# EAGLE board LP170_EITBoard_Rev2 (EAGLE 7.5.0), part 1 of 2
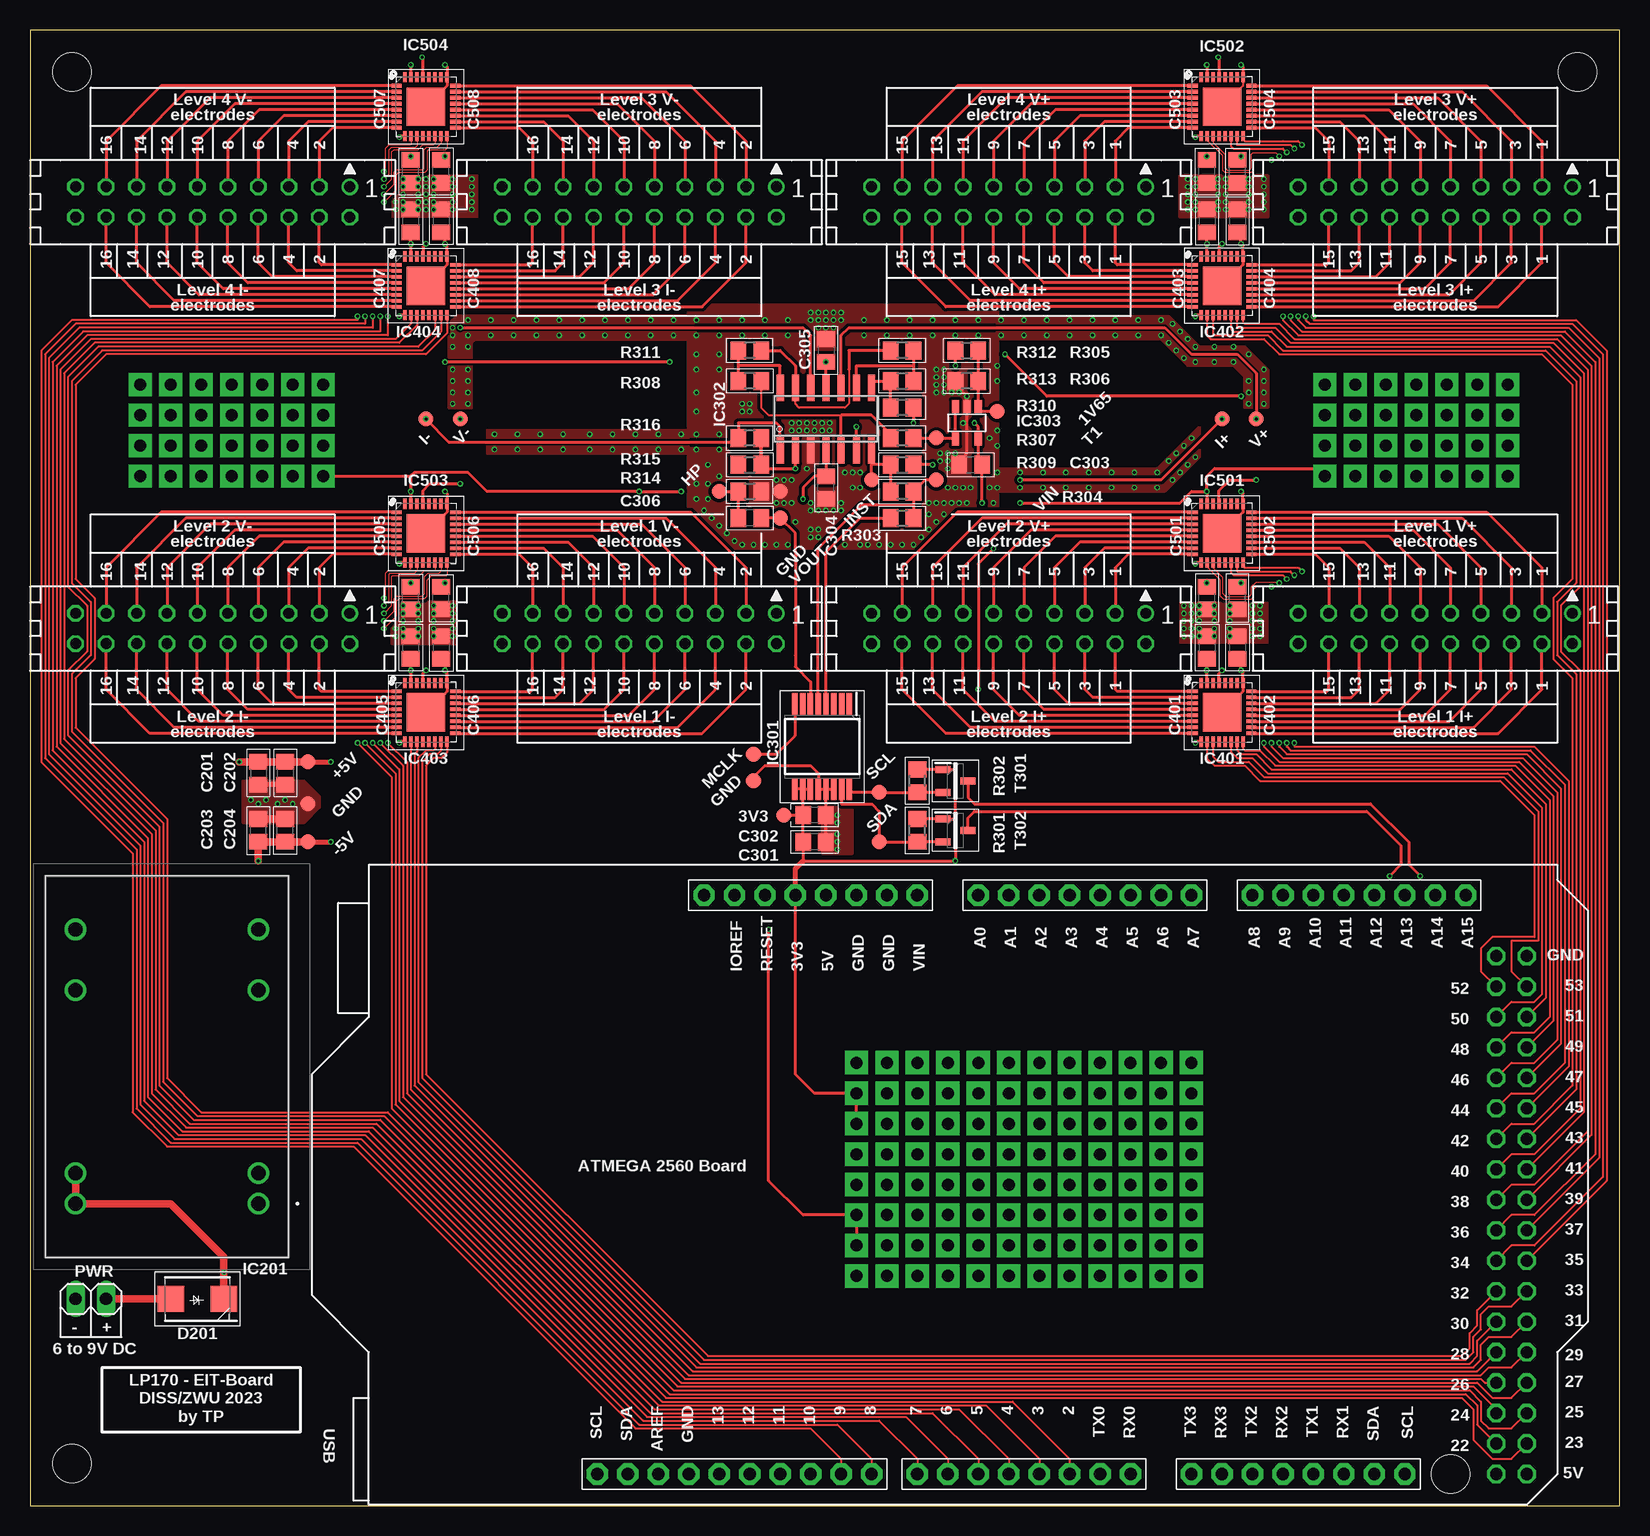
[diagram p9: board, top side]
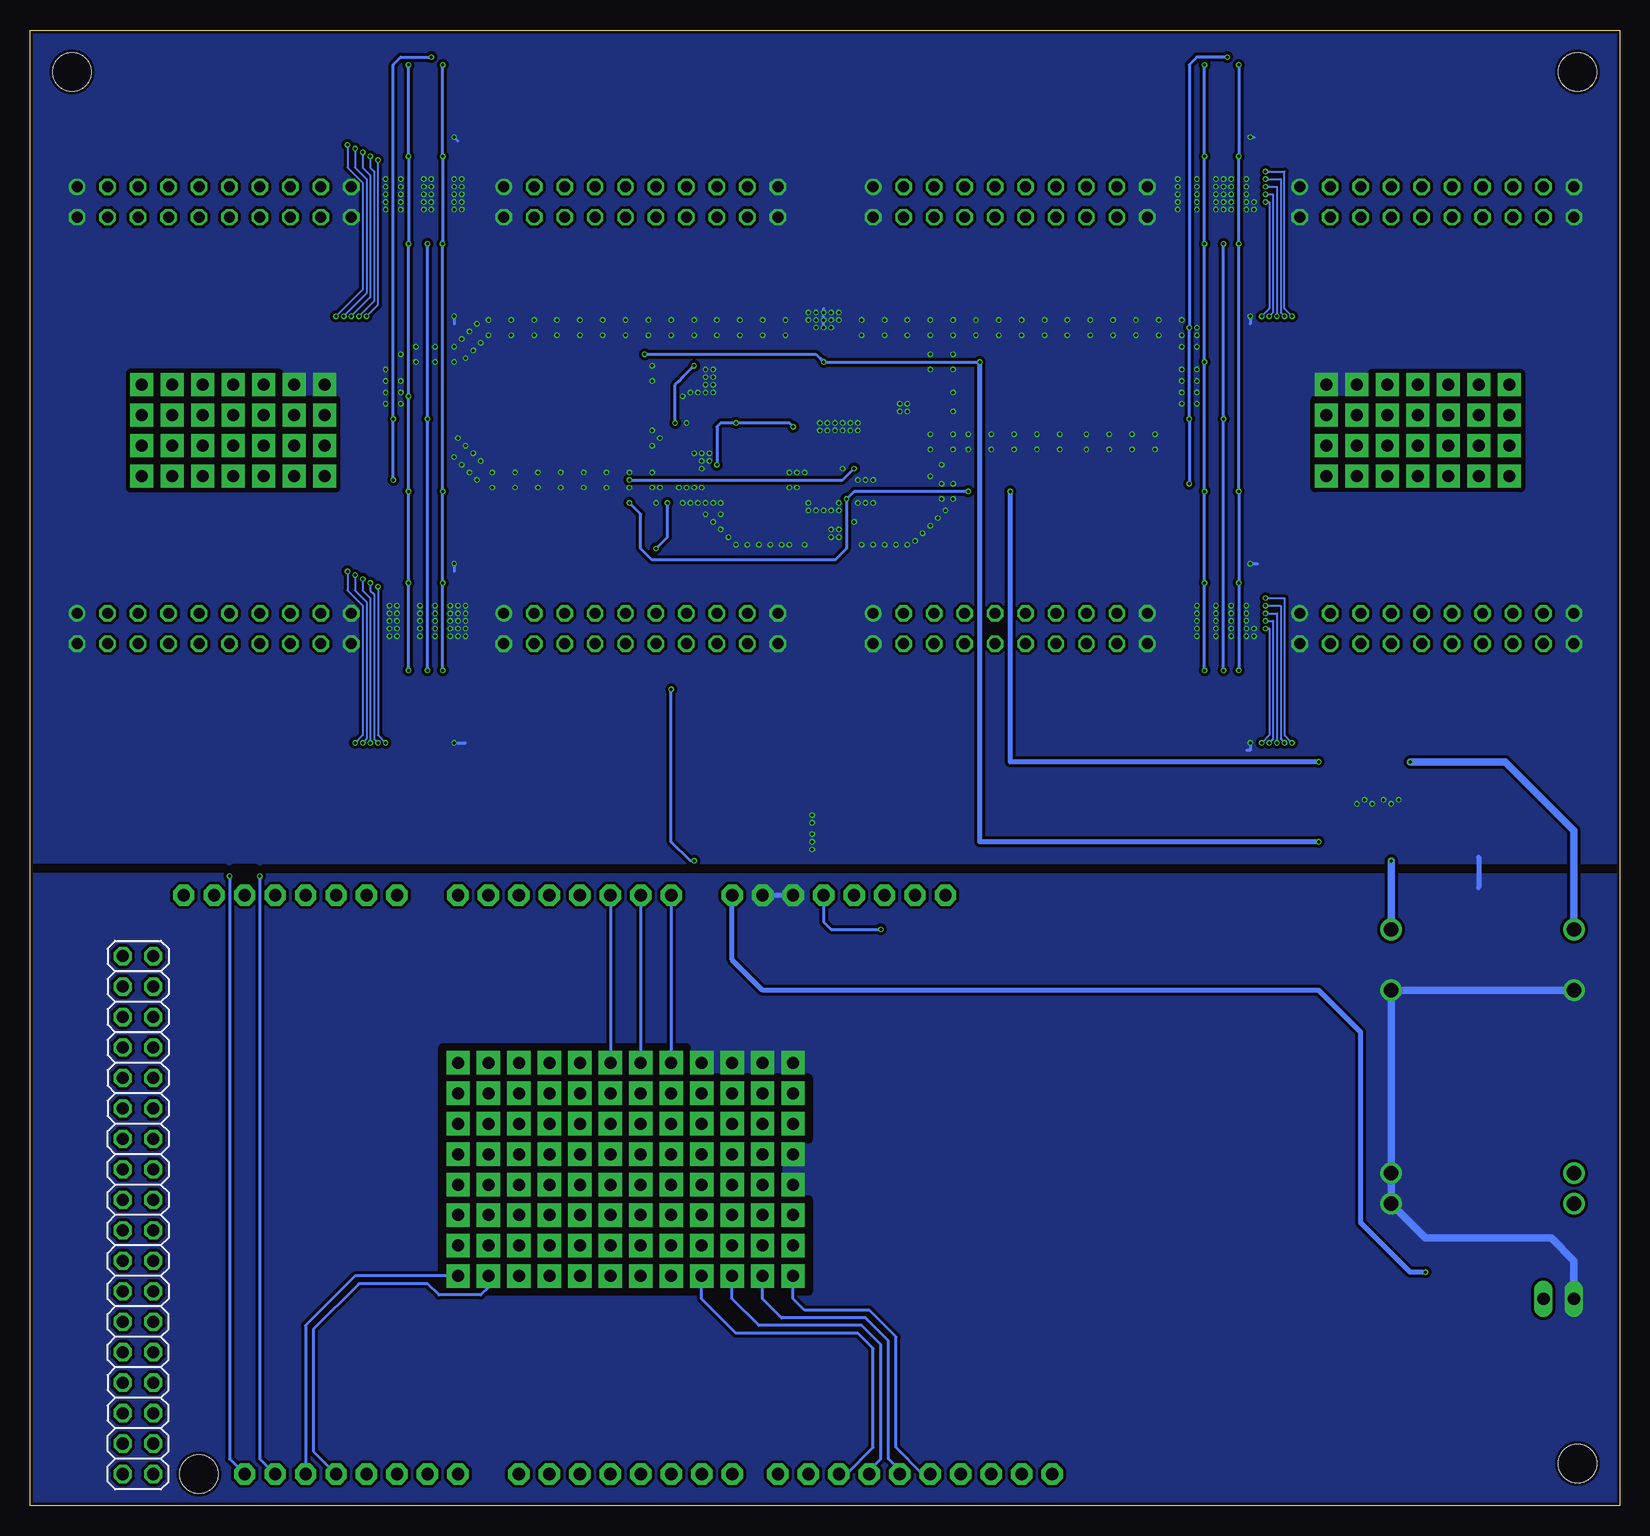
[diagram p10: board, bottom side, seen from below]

Size 132.5 x 123 mm. Coordinates in mm from the lower left corner, seen from the top.
Outline: 0,0 132.5,0 132.5,123 0,123 0,0
Copper layers (1*16): Top 0.018mm / dielectric 1.55mm / Bottom 0.018mm
Design rules "Multi-CB_2L_100µm-Tracks_OL35µm": minimum track width 0.1mm, minimum drill 0.2mm, track to track 0.1mm, track to pad 0.1mm, pad to pad 0.1mm, via to via 0.1mm, smd to smd 0mil, copper to edge 0.2mm, drill to drill 0.2mm, minimum pad ring 0.125mm, minimum via ring 0.1mm, stop-mask expansion 2mil, vias tented up to drill 0.45mm, thermal gap 0.2mm
Holes 3.2 mm at 118.42,2.62 3.5,3.5 3.5,119.5 129,119.5
bRestrict: 27 lines
vRestrict: 1 lines

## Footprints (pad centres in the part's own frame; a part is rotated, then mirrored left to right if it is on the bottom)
B1,27 = smd 1.27 x 1.27: TP 0,0
C0805 = smd 1.3 x 1.5: 1 -0.95,0; 2 0.95,0
CON20 = drill 0.914: 1 -11.43,-1.27 | drill 0.914 octagon: 2 -11.43,1.27; 3 -8.89,-1.27; 4 -8.89,1.27; 5 -6.35,-1.27; 6 -6.35,1.27; 7 -3.81,-1.27; 8 -3.81,1.27; 9 -1.27,-1.27; 10 -1.27,1.27; 11 1.27,-1.27; 12 1.27,1.27; 13 3.81,-1.27; 14 3.81,1.27; 15 6.35,-1.27; 16 6.35,1.27; 17 8.89,-1.27; 18 8.89,1.27; 19 11.43,-1.27; 20 11.43,1.27
DIOM5436X265N = smd 2.2 x 2.15: 1 -2.2,0; 2 2.2,0
DCWN03E15 = drill 1.2 pad 1.8: 2 0,0; 3 0,-2.54; 9 0,-17.78; 11 0,-22.86; 14 15.24,-22.86; 16 15.24,-17.78; 22 15.24,-2.54; 23 15.24,0
SOP65P780X200-16N = smd 1.8 x 0.45: 1 -3.55,2.275; 2 -3.55,1.625; 3 -3.55,0.975; 4 -3.55,0.325; 5 -3.55,-0.325; 6 -3.55,-0.975; 7 -3.55,-1.625; 8 -3.55,-2.275; 9 3.55,-2.275; 10 3.55,-1.625; 11 3.55,-0.975; 12 3.55,-0.325; 13 3.55,0.325; 14 3.55,0.975; 15 3.55,1.625; 16 3.55,2.275
SO14 = smd 0.6 x 2.2: 1 -3.81,-2.6; 2 -2.54,-2.6; 3 -1.27,-2.6; 4 0,-2.6; 5 1.27,-2.6; 6 2.54,-2.6; 7 3.81,-2.6; 8 3.81,2.6; 9 2.54,2.6; 10 1.27,2.6; 11 0,2.6; 12 -1.27,2.6; 13 -2.54,2.6; 14 -3.81,2.6
SOT23-5 = smd 0.6 x 1.2: 1 -0.95,-1.306; 2 0,-1.306; 3 0.95,-1.306; 4 0.95,1.306; 5 -0.95,1.306
QFN50P500X500X80-33N = smd 0.85 x 0.3: 1 -2.45,1.75; 2 -2.45,1.25; 3 -2.45,0.75; 4 -2.45,0.25; 5 -2.45,-0.25; 6 -2.45,-0.75; 7 -2.45,-1.25; 8 -2.45,-1.75; 17 2.45,-1.75; 18 2.45,-1.25; 19 2.45,-0.75; 20 2.45,-0.25; 21 2.45,0.25; 22 2.45,0.75; 23 2.45,1.25; 24 2.45,1.75 | smd 0.3 x 0.85: 9 -1.75,-2.45; 10 -1.25,-2.45; 11 -0.75,-2.45; 12 -0.25,-2.45; 13 0.25,-2.45; 14 0.75,-2.45; 15 1.25,-2.45; 16 1.75,-2.45; 25 1.75,2.45; 26 1.25,2.45; 27 0.75,2.45; 28 0.25,2.45; 29 -0.25,2.45; 30 -0.75,2.45; 31 -1.25,2.45; 32 -1.75,2.45 | smd 3.2 x 3.2: 33 0,0
1X08-BIG = drill 1.016 pad 1.778 octagon: 1 -8.89,0; 2 -6.35,0; 3 -3.81,0; 4 -1.27,0; 5 1.27,0; 6 3.81,0; 7 6.35,0; 8 8.89,0
1X10-BIG = drill 1.016 pad 1.778 octagon: 1 -11.43,0; 2 -8.89,0; 3 -6.35,0; 4 -3.81,0; 5 -1.27,0; 6 1.27,0; 7 3.81,0; 8 6.35,0; 9 8.89,0; 10 11.43,0
2X18 = drill 1.016 octagon: 1 -21.59,-1.27; 2 -21.59,1.27; 3 -19.05,-1.27; 4 -19.05,1.27; 5 -16.51,-1.27; 6 -16.51,1.27; 7 -13.97,-1.27; 8 -13.97,1.27; 9 -11.43,-1.27; 10 -11.43,1.27; 11 -8.89,-1.27; 12 -8.89,1.27; 13 -6.35,-1.27; 14 -6.35,1.27; 15 -3.81,-1.27; 16 -3.81,1.27; 17 -1.27,-1.27; 18 -1.27,1.27; 19 1.27,-1.27; 20 1.27,1.27; 21 3.81,-1.27; 22 3.81,1.27; 23 6.35,-1.27; 24 6.35,1.27; 25 8.89,-1.27; 26 8.89,1.27; 27 11.43,-1.27; 28 11.43,1.27; 29 13.97,-1.27; 30 13.97,1.27; 31 16.51,-1.27; 32 16.51,1.27; 33 19.05,-1.27; 34 19.05,1.27; 35 21.59,-1.27; 36 21.59,1.27
1X02 = drill 1.016 long: 1 -1.27,0; 2 1.27,0
R0805 = smd 1.3 x 1.5: 1 -0.95,0; 2 0.95,0
SOT96P237X111-3N = smd 1.25 x 0.6: 1 -1.05,0.955; 2 -1.05,-0.955; 3 1.05,0

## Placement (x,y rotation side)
1V65  PTR1B1,27  [B1,27]  80.63,91.2 180 top
3V3  PTR1B1,27  [B1,27]  62.85,57.55 0 top
+5V  PTR1B1,27  [B1,27]  23.16,61.99 180 top
-5V  PTR1B1,27  [B1,27]  23.16,55.33 180 top
C201  10u  [C0805]  19.04,61.04 270 top
C202  100n  [C0805]  21.26,61.04 270 top
C203  10u  [C0805]  19.04,56.28 90 top
C204  100n  [C0805]  21.26,56.28 90 top
C301  10u  [C0805]  65.39,55.33 180 top
C302  100n  [C0805]  65.39,57.55 180 top
C303  100n  [C0805]  78.41,86.76 0 top
C304  100n  [C0805]  66.34,84.85 90 top
C305  100n  [C0805]  66.34,96.28 270 top
C306  10n  [C0805]  60,82.31 180 top
C401  100n  [C0805]  98.09,71.52 270 top
C402  100n  [C0805]  100.64,71.52 270 top
C403  100n  [C0805]  98.09,107.08 270 top
C404  100n  [C0805]  100.64,107.08 270 top
C405  100n  [C0805]  31.74,71.52 270 top
C406  100n  [C0805]  34.28,71.52 270 top
C407  100n  [C0805]  31.74,107.08 270 top
C408  100n  [C0805]  34.28,107.08 270 top
C501  100n  [C0805]  98.09,75.64 90 top
C502  100n  [C0805]  100.64,75.64 90 top
C503  100n  [C0805]  98.09,111.2 90 top
C504  100n  [C0805]  100.64,111.2 90 top
C505  100n  [C0805]  31.74,75.64 90 top
C506  100n  [C0805]  34.28,75.64 90 top
C507  100n  [C0805]  31.74,111.2 90 top
C508  100n  [C0805]  34.28,111.2 90 top
CON-LEVEL1-I+/V+  [CON20]  117.14,73.11 180 top
CON-LEVEL1-I-/V-  [CON20]  50.79,73.11 180 top
CON-LEVEL2-I+/V+  [CON20]  81.59,73.11 180 top
CON-LEVEL2-I-/V-  [CON20]  15.23,73.11 180 top
CON-LEVEL3-I+/V+  [CON20]  117.14,108.67 180 top
CON-LEVEL3-I-/V-  [CON20]  50.79,108.67 180 top
CON-LEVEL4-I+/V+  [CON20]  81.59,108.67 180 top
CON-LEVEL4-I-/V-  [CON20]  15.23,108.67 180 top
D201  STPS1L40U  [DIOM5436X265N]  13.96,17.23 180 top
G  PTR1B1,27  [B1,27]  23.16,58.5 180 top
GND  PTR1B1,27  [B1,27]  62.53,84.53 0 top
GND70  PTR1B1,27  [B1,27]  60.31,60.41 0 top
HP  PTR1B1,27  [B1,27]  57.45,84.53 0 top
I+  PTR1B1,27  [B1,27]  99.37,90.57 0 top
I-  PTR1B1,27  [B1,27]  33.01,90.57 0 top
IC201  DCWN03E-5  [DCWN03E15]  19.04,25.16 180 top
IC301  AD5933WYRSZ  [SOP65P780X200-16N]  66.03,63.26 270 top
IC302  TL084QDR  [SO14]  66.34,90.57 0 top
IC303  LMV321M5X  [SOT23-5]  78.09,90.25 180 top
IC401  DG1206ETJ+  [QFN50P500X500X80-33N]  99.37,66.12 0 top
IC402  DG1206ETJ+  [QFN50P500X500X80-33N]  99.37,101.68 0 top
IC403  DG1206ETJ+  [QFN50P500X500X80-33N]  33.01,66.12 0 top
IC404  DG1206ETJ+  [QFN50P500X500X80-33N]  33.01,101.68 0 top
IC501  DG1206ETJ+  [QFN50P500X500X80-33N]  99.37,81.04 0 top
IC502  DG1206ETJ+  [QFN50P500X500X80-33N]  99.37,116.6 0 top
IC503  DG1206ETJ+  [QFN50P500X500X80-33N]  33.01,81.04 0 top
IC504  DG1206ETJ+  [QFN50P500X500X80-33N]  33.01,116.6 0 top
INST  PTR1B1,27  [B1,27]  70.16,85.49 90 top
MCLK  PTR1B1,27  [B1,27]  60.31,62.63 0 top
MEGA_CON1  [1X08-BIG]  65.08,50.88 180 top
MEGA_CON2  [1X08-BIG]  87.94,50.88 180 top
MEGA_CON3  [1X08-BIG]  110.8,50.88 180 top
MEGA_CON4  [1X08-BIG]  105.72,2.62 0 top
MEGA_CON5  [1X08-BIG]  82.85,2.62 0 top
MEGA_CON6  [1X10-BIG]  58.73,2.62 0 top
MEGA_CON7  [2X18]  123.5,24.21 270 bottom
PWR  [1X02]  5.07,17.23 0 top
R301  10k  [R0805]  73.97,56.28 90 top
R302  10k  [R0805]  73.97,60.41 90 top
R303  220k  [R0805]  72.69,82.31 0 top
R304  22k  [R0805]  72.69,84.53 180 top
R305  10k  [R0805]  78.09,96.28 0 top
R306  10k  [R0805]  78.09,93.74 180 top
R307  68k  [R0805]  72.69,88.98 180 top
R308  68k  [R0805]  60,93.74 180 top
R309  68k  [R0805]  72.69,86.76 0 top
R310  68k  [R0805]  72.69,91.52 180 top
R311  27k  [R0805]  60,96.28 180 top
R312  1M  [R0805]  72.69,96.28 180 top
R313  27k  [R0805]  72.69,93.74 0 top
R314  100k  [R0805]  60,84.53 0 top
R315  1k  [R0805]  60,86.76 0 top
R316  10k  [R0805]  60,88.98 180 top
SCL  PTR1B1,27  [B1,27]  70.79,59.45 90 top
SDA  PTR1B1,27  [B1,27]  70.79,55.33 90 top
T1  PTR1B1,27  [B1,27]  75.55,88.98 180 top
T301  BSS138  [SOT96P237X111-3N]  77.14,60.41 0 top
T302  BSS138  [SOT96P237X111-3N]  77.14,56.28 0 top
V+  PTR1B1,27  [B1,27]  102.22,90.57 90 top
V-  PTR1B1,27  [B1,27]  35.87,90.57 90 top
VIN  PTR1B1,27  [B1,27]  75.55,85.49 90 top
VOUT  PTR1B1,27  [B1,27]  62.53,82.31 0 top

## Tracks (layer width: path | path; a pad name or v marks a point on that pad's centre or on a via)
5V_M  (via drill 0.25, 1 pad 1.93)
  Top 0.254: v61.58,48.02 61.58,27.07 64.44,24.21 v68.88,24.21 v68.88,21.67
  Bottom 0.254: MEGA_CON1.4 66.34,48.66 65.71,48.02 v61.58,48.02
+3V3  (via drill 0.25, 1 pad 1.93)
  Top 0.254: C302.2 C301.2 64.44,53.74 v77.14,53.74 77.14,57.55 | IC301.10 IC301.11 | IC301.10 IC301.9 | IC301.10 64.4,57.59 C302.2 | 77.14,57.55 77.14,61.36 T301.1 R302.2 | 77.14,57.55 77.14,57.23 T302.1 R301.2 | v77.14,95.01 R305.1 | v78.73,90.25 79.04,89.94 IC303.5 79.04,86.76 C303.2 79.36,86.44 C303.2 v79.36,83.58 | 3V3.TP C302.2 | v79.05,68.03 79.05,78.5 v80.31,79.77 | v68.88,31.83 v68.88,34.37 65.39,34.37 63.8,35.96 MEGA_CON1.5
  Top 0.406: MEGA_CON1.5 63.8,53.1 64.44,53.74
  Bottom 0.254: v78.73,90.25 78.73,93.42 78.41,93.74 78.09,94.06 v77.14,95.01 | v77.14,53.74 77.46,53.74 79.05,55.33 v79.05,68.03 | v79.36,83.58 79.36,80.72 v80.31,79.77
+5V  (via drill 0.25, 1 pad 1.93)
  Top 0.254: C304.2 | IC401.31 98.12,70.55 C401.2 v98.09,69.61 | C501.2 v98.09,76.92 | v98.09,84.53 98.09,83.51 IC501.31 | IC402.31 v98.12,105.17 98.12,106.11 C403.2 | C503.2 v98.09,112.47 | v98.09,120.09 98.09,119.07 IC502.31 | IC504.31 31.76,120.08 v31.74,120.09 | v31.74,112.47 C507.2 | IC404.31 31.76,105.15 v31.74,105.17 C407.2 | IC503.31 31.76,84.52 v31.74,84.53 31.74,85.81 | v31.74,76.92 C505.2 | C405.2 v31.74,69.61 31.76,69.59 IC403.31 | IC302.4 C304.2 | C304.2 65.39,85.81 64.44,84.85 v64.44,83.9 | v54.28,84.53 v50.79,84.53 38.09,84.53 36.5,86.12 32.05,86.12 31.74,85.81 | v82.54,83.58 95.87,83.58 96.83,84.53 v98.09,84.53 | v98.09,84.53 98.09,85.81 98.73,86.44 107.3,86.44 v107.94,85.81 | v24.44,85.81 31.74,85.81
  Top 0.406: +5V.TP v25.07,61.99
  Top 0.61: +5V.TP C202.1 C201.1 v17.45,61.99
  Bottom 0.254: 98.09,105.47 v98.09,84.53 v98.09,76.92 v98.09,69.61 | 98.09,105.47 v98.12,105.17 | 98.09,105.47 v98.09,112.47 v98.09,120.09 | v31.74,120.09 v31.74,112.47 v31.74,105.17 v31.74,84.53 v31.74,76.92 v31.74,69.61 | v54.28,84.53 63.8,84.53 v64.44,83.9 64.44,79.77 65.39,78.82 80.63,78.82 81.59,79.77 81.59,82.63 v82.54,83.58
  Bottom 0.406: v50.79,84.53 50.79,61.99 v25.07,61.99
  Bottom 0.61: IC201.14 3.8,56.28 9.51,61.99 v17.45,61.99
+5V1  (via drill 1 pad 1.93)
  other vias: 9.2,85.81
+5V2  (via drill 1 pad 1.93)
  other vias: 81.59,19.13
+5V3  (via drill 1 pad 1.93)
  other vias: 81.59,31.83
-5V  (via drill 0.25)
  Top 0.152: IC502.25 101.11,118.35 IC502.33
  Top 0.254: C402.2 101.11,70.09 100.95,69.92 v100.95,69.61 101.11,69.45 IC401.25 101.11,67.87 IC401.33 | IC501.33 101.11,82.79 IC501.25 101.11,84.37 v100.95,84.53 | C502.2 v100.95,76.92 | 101.11,105.65 C404.2 | IC402.33 101.11,103.43 IC402.25 101.11,105.01 v100.95,105.17 100.95,105.81 C404.2 | C404.2 100.95,106.13 100.95,106.12 | C504.2 v100.95,112.47 | v100.95,120.09 101.11,119.93 IC502.25 | v34.59,76.92 C506.2 | C406.2 34.59,70.25 v34.59,69.61 34.76,69.45 IC403.25 34.76,67.87 IC403.33 | IC404.33 34.76,103.43 IC404.25 34.76,105.01 v34.59,105.17 34.59,105.81 C408.2 | v34.59,112.47 C508.2 | v34.59,120.09 34.76,119.93 IC504.25 34.76,118.35 IC504.33 | v34.59,84.53 34.76,84.37 IC503.25 34.76,82.79 IC503.33 | IC302.11 C305.2 | v53.33,95.33 v34.59,95.33 | v100.95,92.47 84.76,92.47 v81.27,95.97
  Top 0.406: -5V.TP v25.07,55.33
  Top 0.61: -5V.TP C204.1 C203.1 v19.04,53.74
  Bottom 0.254: v100.95,69.61 v100.95,76.92 v100.95,84.53 v100.95,92.47 v100.95,105.17 v100.95,112.47 v100.95,120.09 | v34.59,69.61 v34.59,76.92 v34.59,84.53 v34.59,95.33 v34.59,105.17 v34.59,112.47 v34.59,120.09 | C305.2 v53.33,95.33 | C305.2 66.66,95.65 | v81.27,95.97 66.98,95.97 C305.2
  Bottom 0.406: v53.33,95.33 53.33,55.33 v25.07,55.33
  Bottom 0.61: IC201.11 v19.04,53.74
  other vias: 66.34,95.33
A0  (via drill 1 pad 1.93)
  Bottom 0.254: MEGA_CON2.8 v79.05,36.91
A0_DEMUX1
  Top 0.152: IC401.15 100.61,62.97 100.95,62.63 102.22,62.63 103.49,61.36 123.5,61.36 126.35,58.5 126.35,42.31 MEGA_CON7.5
A0_DEMUX2
  Top 0.152: IC402.15 100.61,98.21 100.64,98.19 103.81,98.19 105.08,96.92 126.99,96.92 129.53,94.38 129.53,32.78 MEGA_CON7.15
A0_DEMUX3
  Top 0.152: IC403.15 34.26,62.92 33.96,62.63 33.33,62.63 32.69,61.99 32.69,35.64 56.19,12.14 119.69,12.14 120.32,12.78 120.32,14.05 120.95,14.68 120.95,15.95 121.59,16.59 123.5,16.59 MEGA_CON7.23
A0_DEMUX4
  Top 0.152: IC404.15 34.26,97.85 32.69,96.28 6.02,96.28 3.48,93.74 3.48,76.92 5.07,75.33 5.07,70.88 3.48,69.3 3.48,64.53 11.1,56.91 11.1,35.32 13.96,32.47 29.52,32.47 53.01,8.97 119.37,8.97 120.32,8.02 120.32,5.48 121.91,3.89 122.22,3.89 123.5,3.89 MEGA_CON7.33
A0_MUX1  (via drill 0.25)
  Top 0.152: IC501.15 100.61,77.89 100.64,77.87 105.08,77.87 v105.4,77.55 | v104.76,63.58 104.76,63.26 105.08,62.94 125.08,62.94 127.94,60.09 127.94,36.91 125.4,34.37 123.5,34.37 MEGA_CON7.12
  Bottom 0.152: v105.4,77.55 105.4,76.28 104.44,75.33 104.44,63.9 v104.76,63.58
A0_MUX2  (via drill 0.25)
  Top 0.152: IC502.15 100.61,113.45 100.64,113.43 103.81,113.43 105.08,113.43 v105.4,113.11 | v106.35,99.14 106.35,98.82 106.67,98.5 128.57,98.5 131.12,95.97 131.12,27.38 125.4,21.67 123.5,21.67 MEGA_CON7.22
  Bottom 0.152: v105.4,113.11 105.4,111.52 104.44,110.57 104.44,101.05 v106.35,99.14
A0_MUX3  (via drill 0.25)
  Top 0.102: IC503.15 34.26,77.9 34.06,77.7 33.15,77.7 32.84,77.4 32.84,75.97 32.64,75.77 30.51,75.77 30.3,75.57 30.3,74.53 v29.52,73.74
  Top 0.152: v29.2,63.58 31.1,61.67 31.1,34.05 54.6,10.56 120.95,10.56 121.27,10.24 MEGA_CON7.30
  Bottom 0.152: v29.52,73.74 28.88,73.74 28.88,63.9 v29.2,63.58
A0_MUX4  (via drill 0.25)
  Top 0.1: 34.26,113.56 33.9,113.2 33,113.2 32.8,113 | 32.8,111.4 32.7,111.3 30.5,111.3 30.3,111.1 30.3,110.08 v29.52,109.3
  Top 0.102: IC504.15 34.26,113.56 | 32.8,113 32.8,111.4
  Top 0.152: v29.2,99.14 29.2,97.87 4.43,97.87 1.89,95.33 1.89,62.94 9.51,55.33 9.51,33.73 12.37,30.88 27.93,30.88 51.42,7.38 73.01,7.38 76.5,3.89 MEGA_CON5.2
  Bottom 0.152: v29.52,109.3 28.88,109.3 28.88,99.46 v29.2,99.14
A1  (via drill 1 pad 1.93)
  Bottom 0.254: MEGA_CON2.7 v81.59,36.91
A1_DEMUX1
  Top 0.152: IC401.14 100.12,62.83 100.64,62.31 101.91,62.31 103.17,61.04 123.18,61.04 126.03,58.18 126.03,42.62 125.4,41.99 123.5,41.99 MEGA_CON7.6
A1_DEMUX2
  Top 0.152: IC402.14 100.12,98.07 100.32,97.87 103.49,97.87 104.76,96.6 126.67,96.6 129.21,94.06 129.21,76.6 127.62,75.01 127.62,71.2 129.21,69.61 129.21,33.1 125.4,29.29 123.5,29.29 MEGA_CON7.16
A1_DEMUX3
  Top 0.152: IC403.14 33.76,63.06 33.64,62.94 33.01,62.94 32.37,62.31 32.37,35.32 55.87,11.83 120,11.83 120.64,12.46 120.64,13.73 MEGA_CON7.26
A1_DEMUX4
  Top 0.152: IC404.14 33.76,97.98 32.37,96.6 5.7,96.6 3.16,94.06 3.16,76.6 4.75,75.01 4.75,71.2 3.16,69.61 3.16,64.22 10.78,56.59 10.78,35.01 13.64,32.15 29.2,32.15 52.69,8.65 81.9,8.65 86.66,3.89 MEGA_CON5.6
A1_MUX1  (via drill 0.25)
  Top 0.152: IC501.14 100.12,77.75 100.32,77.55 104.44,77.55 v104.76,77.23 | v104.13,63.58 104.13,63.26 104.76,62.63 124.77,62.63 127.62,59.77 127.62,38.5 MEGA_CON7.9
  Bottom 0.152: v104.76,77.23 104.76,76.28 104.13,75.64 v104.13,63.58
A1_MUX2  (via drill 0.25)
  Top 0.152: IC502.14 100.12,113.31 100.32,113.11 104.44,113.11 v104.76,112.79 | v105.72,99.14 105.72,98.82 106.35,98.19 128.26,98.19 130.8,95.65 130.8,28.97 MEGA_CON7.19
  Bottom 0.152: v104.76,112.79 104.76,111.52 104.13,110.89 104.13,100.73 v105.72,99.14
A1_MUX3  (via drill 0.25)
  Top 0.102: IC503.14 33.76,77.91 | 33.76,77.91 | 33.76,77.91 32.84,77.91 32.44,77.5 30.2,77.5 30.1,77.4 30.1,74.96 v29.52,74.38
  Top 0.152: v28.56,63.58 30.79,61.36 30.79,33.73 54.28,10.24 120.64,10.24 121.91,8.97 123.5,8.97 MEGA_CON7.29
  Bottom 0.152: v29.52,74.38 28.56,74.38 v28.56,63.58
A1_MUX4  (via drill 0.25)
  Top 0.1: 33.76,113.56 33.6,113.4 32.7,113.4 32.3,113 30.3,113 30.1,112.8 30.1,110.52 v29.52,109.94
  Top 0.102: IC504.14 33.76,113.56
  Top 0.152: v28.56,99.14 28.56,98.19 4.12,98.19 1.58,95.65 1.58,62.63 9.2,55.01 9.2,33.42 12.05,30.56 27.61,30.56 51.11,7.06 70.79,7.06 73.97,3.89 MEGA_CON5.1
  Bottom 0.152: v29.52,109.94 28.56,109.94 v28.56,99.14
A2  (via drill 1 pad 1.93)
  Bottom 0.254: MEGA_CON2.6 v84.12,36.91
A2_DEMUX1
  Top 0.152: IC401.11 98.62,62.42 99.05,61.99 101.59,61.99 102.86,60.72 122.86,60.72 125.72,57.87 125.72,47.07 123.5,47.07 123.5,44.53 MEGA_CON7.3
A2_DEMUX2
  Top 0.152: IC402.11 98.62,97.67 98.73,97.55 103.17,97.55 104.44,96.28 126.35,96.28 128.89,93.74 128.89,76.92 127.31,75.33 127.31,70.88 128.89,69.3 128.89,34.69 MEGA_CON7.13
A2_DEMUX3
  Top 0.152: IC403.11 32.26,62.83 32.05,62.63 32.05,35.01 55.55,11.51 120.32,11.51 120.95,12.14 120.95,13.41 121.59,14.05 123.5,14.05 MEGA_CON7.25
A2_DEMUX4
  Top 0.152: IC404.11 32.26,98.39 30.79,96.92 5.39,96.92 2.84,94.38 2.84,63.9 10.46,56.28 10.46,34.69 13.32,31.83 28.88,31.83 52.38,8.34 79.68,8.34 84.12,3.89 MEGA_CON5.5
A2_MUX1  (via drill 0.25)
  Top 0.102: IC501.11 98.62,78.17 99.39,77.4 99.39,76.08 99.69,75.77 101.63,75.77 101.83,75.97 101.83,76.58 102.23,76.99 104.05,76.99 v104.13,76.92
  Top 0.152: v103.49,63.58 103.49,63.26 104.44,62.31 124.45,62.31 127.31,59.45 127.31,38.81 125.4,36.91 123.5,36.91 MEGA_CON7.10
  Bottom 0.152: v104.13,76.92 104.13,76.28 103.81,75.96 103.81,63.9 v103.49,63.58
A2_MUX2  (via drill 0.25)
  Top 0.102: IC502.11 98.62,113.63 99.59,112.65 99.59,111.53 99.8,111.33 101.63,111.33 101.83,111.53 101.83,112.65 101.93,112.75 103.85,112.75 v104.13,112.47
  Top 0.152: v105.08,99.14 105.08,98.82 106.03,97.87 127.94,97.87 130.48,95.33 130.48,29.29 125.4,24.21 123.5,24.21 MEGA_CON7.20
  Bottom 0.152: v104.13,112.47 104.13,111.52 103.81,111.2 103.81,100.41 v105.08,99.14
A2_MUX3  (via drill 0.25)
  Top 0.102: IC503.11 32.26,77.93 32.03,77.7 30,77.7 29.9,77.6 29.9,75.39 v29.52,75.01
  Top 0.152: v27.93,63.58 30.47,61.04 30.47,33.42 53.96,9.92 120.32,9.92 122.22,8.02 MEGA_CON7.32
  Bottom 0.152: v29.52,75.01 28.24,75.01 28.24,63.9 v27.93,63.58
A2_MUX4  (via drill 0.25)
  Top 0.1: 32.26,113.36 32.1,113.2 30.1,113.2 29.9,113 29.9,110.95 v29.52,110.57
  Top 0.102: IC504.11 32.26,113.36
  Top 0.152: v27.93,99.14 27.93,98.5 3.8,98.5 1.26,95.97 1.26,62.31 8.88,54.69 8.88,33.1 11.73,30.24 27.29,30.24 50.79,6.75 67.3,6.75 70.16,3.89 MEGA_CON6.10
  Bottom 0.152: v29.52,110.57 28.24,110.57 28.24,99.46 v27.93,99.14
A3_DEMUX1
  Top 0.152: IC401.10 98.12,62.29 98.73,61.67 101.27,61.67 102.54,60.41 122.54,60.41 125.4,57.55 125.4,47.39 121.91,47.39 120.95,46.44 120.95,44.53 MEGA_CON7.4
A3_DEMUX2
  Top 0.152: IC402.10 98.12,97.53 98.41,97.23 102.86,97.23 104.13,95.97 126.03,95.97 128.57,93.42 128.57,77.23 126.99,75.64 126.99,70.56 128.57,68.98 128.57,35.01 125.4,31.83 123.5,31.83 MEGA_CON7.14
A3_DEMUX3
  Top 0.152: IC403.10 31.76,62.97 31.74,62.94 31.74,34.69 55.23,11.19 120.64,11.19 MEGA_CON7.28
A3_DEMUX4
  Top 0.152: IC404.10 31.76,98.53 30.47,97.23 5.07,97.23 2.53,94.69 2.53,63.58 10.15,55.96 10.15,34.37 13,31.51 28.56,31.51 52.06,8.02 77.46,8.02 81.59,3.89 MEGA_CON5.4
A3_MUX1  (via drill 0.25)
  Top 0.102: IC501.10 98.12,78.27 99.19,77.19 99.19,75.87 99.49,75.57 101.83,75.57 102.03,75.77 102.03,76.38 102.23,76.58 103.48,76.58 v103.49,76.6
  Top 0.152: v102.86,63.58 102.86,63.26 104.13,61.99 124.13,61.99 126.99,59.14 126.99,40.4 MEGA_CON7.7
  Bottom 0.152: v103.49,76.6 103.49,64.22 v102.86,63.58
A3_MUX2  (via drill 0.25)
  Top 0.102: IC502.10 98.12,113.83 99.39,112.55 99.39,111.33 99.59,111.13 101.83,111.13 102.03,111.33 102.03,112.04 102.23,112.25 103.4,112.25 v103.49,112.16
  Top 0.152: v104.44,99.14 104.44,98.82 105.72,97.55 127.62,97.55 130.16,95.01 130.16,30.88 MEGA_CON7.17
  Bottom 0.152: v103.49,112.16 103.49,100.09 v104.44,99.14
A3_MUX3  (via drill 0.25)
  Top 0.102: 31.74,78.57 31.74,78.12 31.52,77.91 29.79,77.91 29.59,77.7 29.59,75.72 v29.52,75.64
  Top 0.152: IC503.10 31.74,78.57 | v27.29,63.58 30.15,60.72 30.15,33.1 53.64,9.61 120,9.61 120.95,8.65 120.95,7.06 121.59,6.43 123.5,6.43 MEGA_CON7.31
  Bottom 0.152: v29.52,75.64 27.93,75.64 27.93,64.22 v27.29,63.58
A3_MUX4  (via drill 0.25)
  Top 0.1: IC504.10 31.76,113.46 31.7,113.4 29.9,113.4 29.6,113.1 | 29.6,111.29 v29.52,111.2
  Top 0.102: 29.6,113.1 29.6,111.29
  Top 0.152: v27.29,99.14 27.29,98.82 3.48,98.82 0.94,96.28 0.94,61.99 8.56,54.37 8.56,32.78 11.42,29.92 26.98,29.92 50.47,6.43 65.08,6.43 67.61,3.89 MEGA_CON6.9
  Bottom 0.152: v29.52,111.2 27.93,111.2 27.93,99.78 v27.29,99.14
D10  (via drill 1 pad 1.93)
  Bottom 0.254: MEGA_CON6.8 64.44,2.62 62.22,4.84 62.22,13.1 63.49,14.37 73.65,14.37 76.5,17.23 v76.5,19.13
D11  (via drill 1 pad 1.93)
  Bottom 0.254: MEGA_CON6.7 62.53,2.94 61.58,3.89 61.58,13.41 63.17,15 71.74,15 73.97,17.23 v73.97,19.13
D12  (via drill 1 pad 1.93)
  Bottom 0.254: MEGA_CON6.6 60,2.94 60.95,3.89 60.95,13.73 62.85,15.64 69.84,15.64 71.42,17.23 v71.42,19.13
D13  (via drill 1 pad 1.93)
  Bottom 0.254: MEGA_CON6.5 58.09,2.62 60.31,4.84 60.31,14.05 62.53,16.27 67.93,16.27 68.88,17.23 v68.88,19.13
EN_DEMUX1
  Top 0.152: IC401.16 101.11,63.1 101.27,62.94 102.54,62.94 103.81,61.67 123.81,61.67 126.67,58.82 126.67,40.72 125.4,39.45 123.5,39.45 MEGA_CON7.8
EN_DEMUX2
  Top 0.152: IC402.16 101.11,98.66 101.27,98.5 104.13,98.5 105.4,97.23 127.31,97.23 129.84,94.69 129.84,31.2 125.4,26.75 123.5,26.75 MEGA_CON7.18
EN_DEMUX3
  Top 0.152: IC403.16 34.76,62.79 34.28,62.31 33.64,62.31 33.01,61.67 33.01,35.96 56.5,12.46 119.37,12.46 120,13.1 120,14.37 120.64,15 120.64,16.27 MEGA_CON7.24
EN_DEMUX4
  Top 0.152: IC404.16 34.76,97.72 33.01,95.97 6.34,95.97 3.8,93.42 3.8,77.23 5.39,75.64 5.39,70.56 3.8,68.98 3.8,64.85 11.42,57.23 11.42,35.64 14.27,32.78 29.83,32.78 53.33,9.29 119.69,9.29 120.64,8.34 120.64,6.75 120.95,6.43 MEGA_CON7.34
EN_MUX1  (via drill 0.25)
  Top 0.152: IC501.16 101.11,78.34 101.27,78.19 105.72,78.19 v106.03,77.87 | v105.4,63.58 105.4,63.26 125.4,63.26 128.26,60.41 128.26,36.59 MEGA_CON7.11
  Bottom 0.152: v106.03,77.87 106.03,76.28 104.76,75.01 104.76,64.22 v105.4,63.58
EN_MUX2  (via drill 0.25)
  Top 0.152: IC502.16 101.11,113.9 101.27,113.75 104.44,113.75 105.72,113.75 v106.03,113.43 | v106.98,99.14 106.98,98.82 128.89,98.82 131.43,96.28 131.43,27.07 MEGA_CON7.21
  Bottom 0.152: v106.03,113.43 106.03,111.52 104.76,110.25 104.76,101.36 v106.98,99.14
EN_MUX3  (via drill 0.25)
  Top 0.102: IC503.16 34.76,77.58 34.67,77.5 33.45,77.5 33.05,77.09 33.05,75.77 32.84,75.57 30.71,75.57 30.51,75.37 30.51,74.1 v29.52,73.11
  Top 0.152: v29.83,63.58 31.42,61.99 31.42,34.37 54.91,10.88 120.95,10.88 121.59,11.51 123.5,11.51 MEGA_CON7.27
  Bottom 0.152: v29.52,73.11 29.2,73.11 29.2,64.22 v29.83,63.58
EN_MUX4  (via drill 0.25)
  Top 0.1: IC504.16 34.76,113.16 34.6,113 33.2,113 33.1,112.9 | 33.1,111.3 32.9,111.1 30.7,111.1 30.5,110.9 30.5,109.65 v29.52,108.67
  Top 0.102: 33.1,112.9 33.1,111.3
  Top 0.152: v29.83,99.14 29.83,97.55 4.75,97.55 2.21,95.01 2.21,63.26 9.83,55.64 9.83,34.05 12.69,31.2 28.24,31.2 51.74,7.7 75.23,7.7 79.05,3.89 MEGA_CON5.3
  Bottom 0.152: v29.52,108.67 29.2,108.67 29.2,99.78 v29.83,99.14
GND  (via drill 0.25, 1 pad 1.93)
  Top 0.254: C301.1 C302.1 IC301.13 | IC301.13 IC301.12 65.71,61.04 65.08,61.67 61.27,61.67 60.31,60.72 GND70.TP | IC301.13 IC301.14 | R306.2 77.46,93.43 77.46,93.11 v78.09,92.47 IC303.2 78.09,87.71 77.46,87.08 C303.1 | IC504.9 30.88,114.15 v30.79,114.06 | v31.1,110.57 C507.1 | v31.1,108.03 C407.1 | C508.1 33.96,110.25 v35.23,110.57 | C408.1 v33.64,108.03 v35.23,108.03 | IC404.9 30.88,99.23 v30.79,99.14 | IC502.9 97.23,114.15 v97.14,114.06 | IC503.9 30.88,78.59 v30.79,78.5 | IC403.9 30.88,63.67 v30.79,63.58 | IC501.9 97.23,78.59 v97.14,78.5 | IC402.9 97.23,99.23 v97.14,99.14 | C305.1 v66.34,98.19 | IC401.9 97.23,63.67 v97.14,63.58
  Top 0.406: C202.2 C201.2
  Top 0.61: C203.2 C204.2
  Bottom 0.254: v30.79,114.06 30.47,114.06 | v30.79,99.14 30.79,98.5 | v97.14,114.06 96.83,113.75 | v30.79,78.5 30.15,78.5 | v30.79,63.58 30.79,62.94 31.1,62.94 | v97.14,78.5 97.14,77.87 | v97.14,99.14 97.14,98.5 | v66.34,98.19 66.34,99.78 | v97.14,63.58 96.19,63.58
  Bottom 0.406: MEGA_CON1.2 MEGA_CON1.3 | 11.73,54.05 11.73,51.52
  Bottom 0.61: PWR.1 3.8,20.4 5.7,22.3 16.18,22.3 IC201.2 IC201.3 IC201.9 IC201.16
  other vias: 18.4,58.82 19.04,58.5 19.67,58.82 20.62,58.5 21.26,58.82 21.89,58.5 67.3,57.55 67.3,55.33 67.3,55.96 67.3,54.69 67.3,56.91 32.37,110.57 33.64,109.94 32.37,108.67 33.64,108.67 35.23,108.67 31.1,109.3 31.1,108.67 33.01,108.67 33.01,108.03 32.37,108.03 31.1,109.94 32.37,109.94 33.64,110.57 30.47,72.47 31.1,72.47 31.1,73.11 32.37,72.47 33.64,73.74 33.64,73.11 33.64,72.47 35.23,73.11 35.23,72.47 31.1,75.01 31.1,74.38 32.37,75.01 32.37,74.38 33.64,75.01 33.64,74.38 102.86,110.57 102.86,109.94 101.59,110.57 101.59,109.94 99.68,109.3 99.68,108.67 99.05,109.3 99.05,108.67 97.14,108.67 97.14,108.03 96.51,108.67 96.51,108.03 96.51,110.57 96.51,109.94 97.14,110.57 97.14,109.94 99.68,110.57 99.68,109.94 36.82,108.67 36.82,108.03 36.82,109.3 33.01,109.3 33.01,109.94 33.01,110.57 32.37,109.3 33.64,109.3 35.23,109.94 35.23,109.3 36.82,109.94 36.82,110.57 30.47,108.67 30.47,108.03 31.1,73.77 32.37,73.11 32.37,73.74 30.47,73.11 35.23,73.74 35.23,74.38 35.23,75.01 96.51,109.3 97.14,109.3 99.05,110.57 99.05,109.94 99.05,108.03 99.68,108.03 101.59,109.3 101.59,108.67 101.59,108.03 102.86,108.03 102.86,108.67 102.86,109.3 96.19,75.01 96.83,75.01 97.46,75.01 96.19,74.38 96.19,73.74 96.19,73.11 96.19,72.47 96.83,72.47 96.83,73.11 96.83,73.74 96.83,74.38 97.46,74.38 97.46,73.74 97.46,73.11 97.46,72.47 98.73,75.01 98.73,74.38 98.73,73.74 98.73,73.11 98.73,72.47 100,75.01 100,74.38 100,73.74 100,73.11 100,72.47 101.91,75.01 101.91,74.38 101.91,73.74 101.91,73.11 101.91,72.47 102.54,72.47 102.54,73.11 102.54,73.74 102.54,74.38 102.54,75.01 65.71,98.19 66.98,98.19 65.71,98.82 65.71,99.46 65.08,99.46 65.08,98.82 66.34,98.82 66.34,99.46 66.98,98.82 66.98,99.46 67.61,99.46 67.61,98.82 64.76,89.61 65.39,89.61 64.76,90.25 65.39,90.25 64.12,90.25 64.12,89.61 63.49,89.61 63.49,90.25 66.03,90.25 66.03,89.61 66.66,89.61 66.66,90.25 76.5,87.71 75.87,87.71 75.87,87.08 76.5,87.08 76.5,86.44 77.14,87.71 76.19,83.58 77.78,90.25 77.46,92.79 76.82,92.79 76.19,92.79 75.55,92.79 75.55,93.42 75.55,94.06 75.55,94.69 76.19,94.69 76.19,94.06 76.19,93.42 65.71,82.95 66.34,82.95 66.98,82.95 67.61,82.95 67.61,83.58 65.08,82.95 65.08,83.58 62.22,85.49 62.85,85.49 63.49,85.49 62.22,83.58 62.85,83.58 63.49,83.58 67.93,86.12 68.57,86.12 69.2,86.12 74.92,83.58 75.55,83.58 76.82,83.58 77.46,83.58 78.09,83.58 74.92,82.63 55.55,98.82 57.45,98.82 59.36,98.82 61.27,98.82 63.17,98.82 59.36,97.55 61.27,97.55 63.17,97.55 57.45,97.55 55.55,97.55 55.55,95.97 57.45,95.97 55.55,94.69 57.45,94.69 55.55,89.3 57.45,89.3 55.55,88.03 57.45,88.03 55.55,85.17 57.45,85.81 56.5,86.76 55.55,92.79 55.55,91.2 60,91.84 59.36,91.84 59.36,91.2 60,91.2 56.5,85.17 55.55,83.9 56.5,83.9 56.19,82.95 56.82,82.31 57.45,81.68 58.09,81.04 58.73,80.41 59.36,80.09 60.31,80.09 61.27,80.09 62.22,80.09 63.17,80.09 67.93,80.09 69.2,80.09 69.84,80.09 70.79,80.09 71.74,80.09 72.69,80.09 73.65,80.09 74.28,80.72 74.92,81.36 75.55,82 76.19,82.63 65.71,81.36 63.8,82 65.08,80.72 65.08,81.36 65.71,80.72 69.52,98.82 71.42,98.82 73.33,98.82 75.23,98.82 77.14,98.82 79.05,98.82 80.95,98.82 69.52,97.55 71.42,97.55 73.33,97.55 75.23,97.55 77.14,97.55 79.05,97.55 80.95,97.55 80.63,95.01 80.63,93.74 80.63,89.61 80.63,88.34 80,88.98 80.31,83.58 64.76,86.44 68.57,84.85 69.2,84.85 76.5,84.85 77.14,84.85 77.78,84.85 78.41,84.85 80,84.85 80.63,84.85 82.85,98.82 84.76,98.82 86.66,98.82 88.57,98.82 90.47,98.82 92.38,98.82 94.28,98.82 82.85,97.55 84.76,97.55 86.66,97.55 88.57,97.55 90.47,97.55 92.38,97.55 94.28,97.55 94.92,96.92 95.56,96.28 96.19,95.65 95.24,98.5 95.87,97.87 96.51,97.23 97.14,96.6 97.14,95.33 98.73,95.33 98.73,96.6 100.32,96.6 100.32,95.33 101.59,95.97 101.59,93.74 102.86,94.69 102.86,93.74 102.86,92.79 102.86,91.84 101.59,92.79 101.59,91.84 46.02,98.82 47.93,98.82 49.84,98.82 51.74,98.82 53.64,98.82 36.5,98.82 38.41,98.82 40.31,98.82 42.22,98.82 44.12,98.82 35.23,98.19 35.23,97.55 35.23,96.6 35.23,94.69 35.23,93.74 35.23,92.79 35.23,91.84 46.02,97.55 47.93,97.55 49.84,97.55 51.74,97.55 53.64,97.55 36.5,97.55 38.41,97.55 40.31,97.55 42.22,97.55 44.12,97.55 36.5,96.6 36.5,94.69 36.5,93.74 36.5,92.79 36.5,91.84 38.72,89.3 40.63,89.3 42.53,89.3 44.44,89.3 46.66,89.3 48.56,89.3 50.47,89.3 52.38,89.3 54.28,89.3 38.72,88.03 40.63,88.03 42.53,88.03 44.44,88.03 46.66,88.03 48.56,88.03 50.47,88.03 52.38,88.03 54.28,88.03 80.63,86.12 82.54,86.12 84.44,86.12 86.35,86.12 88.25,86.12 82.54,84.85 84.44,84.85 86.35,84.85 88.25,84.85 90.16,84.85 90.16,86.12 92.06,86.12 93.97,86.12 94.92,87.08 92.06,84.85 93.97,84.85 95.24,85.49 95.87,86.12 96.51,86.76 97.14,87.39 95.56,87.71 96.19,88.34 96.83,88.98 107.94,93.42 110.48,93.42 21.89,93.42 24.44,93.42 76.5,36.91 73.97,36.91 71.42,36.91 68.88,36.91 68.88,29.29 68.88,26.75
  pour Bottom (isolate 0.254, no thermals): -0.33,123.27 133.02,123.27 133.02,-0.55 -0.33,-0.55
  pour Top (isolate 0.254, no thermals): 17.77,60.41 22.85,60.41 24.12,59.14 24.12,58.18 22.85,56.91 17.77,56.91
  pour Top (isolate 0.254, no thermals): 66.03,58.18 66.03,54.37 68.57,54.37 68.57,58.18
  pour Top (isolate 0.254, no thermals): 30.15,107.39 37.35,107.39 37.35,110.89 30.15,110.89
  pour Top (isolate 0.254, no thermals): 30.15,71.83 35.55,71.83 35.55,75.33 30.15,75.33
  pour Top (isolate 0.254, no thermals): 95.87,110.89 103.17,110.89 103.17,107.39 95.87,107.39
  pour Top (isolate 0.254, no thermals): 95.87,75.33 103.17,75.33 103.17,71.83 95.87,71.83
  pour Top (isolate 0.254, no thermals): 65.08,97.87 67.61,97.87 67.93,98.5 67.93,99.78 64.76,99.78 64.76,98.5
  pour Top (isolate 0.254, no thermals): 54.91,100.09 80.63,100.09 80.63,79.77 54.91,79.77
  pour Top (isolate 0.152, no thermals): 80.63,99.14 94.92,99.14 97.46,96.6 101.27,96.6 103.17,94.69 103.17,91.52 101.27,91.52 101.27,94.06 100.32,95.01 96.51,95.01 94.28,97.23 80.63,97.23
  pour Top (isolate 0.152, no thermals): 55.23,99.14 35.55,99.14 34.91,98.5 34.91,91.52 36.82,91.52 36.82,96.92 37.13,97.23 55.55,97.23
  pour Top (isolate 0.152, no thermals): 54.91,89.61 38.09,89.61 38.09,87.71 54.91,87.71
  pour Top (isolate 0.254, no thermals): 80.63,86.44 93.97,86.44 97.46,89.93 97.46,87.39 94.92,84.85 94.6,84.53 80.63,84.53
I+  (via drill 0.25)
  Top 0.254: R315.2 R316.1 R315.2 61.27,86.44 v63.8,86.44 IC302.2 | IC401.29 99.12,69.36 v99.37,69.61 | v99.37,105.17 99.12,104.92 IC402.29 | I+.TP 94.28,85.49 v82.54,85.49
  Bottom 0.254: v99.37,69.61 I+.TP v99.37,105.17 | v82.54,85.49 64.76,85.49 v63.8,86.44
  other vias: 99.37,90.57
I+1_1
  Top 0.254: IC401.17 122.38,64.37 126.03,68.03 CON-LEVEL1-I+/V+.4
I+1_2
  Top 0.254: IC401.1 90.63,67.87 90.47,68.03 CON-LEVEL2-I+/V+.4
I+1_3
  Top 0.254: IC402.17 122.38,99.93 126.03,103.58 CON-LEVEL3-I+/V+.4
I+1_4
  Top 0.254: IC402.1 90.63,103.43 90.47,103.58 CON-LEVEL4-I+/V+.4
I+3_1
  Top 0.254: IC401.18 120.34,64.87 123.5,68.03 CON-LEVEL1-I+/V+.6
I+3_2
  Top 0.254: IC401.2 88.59,67.37 87.94,68.03 CON-LEVEL2-I+/V+.6
I+3_3
  Top 0.254: IC402.18 120.34,100.43 123.5,103.58 CON-LEVEL3-I+/V+.6
I+3_4
  Top 0.254: IC402.2 88.59,102.93 87.94,103.58 CON-LEVEL4-I+/V+.6
I+5_1
  Top 0.254: IC401.19 118.3,65.37 120.95,68.03 CON-LEVEL1-I+/V+.8
I+5_2
  Top 0.254: IC401.3 86.55,66.87 85.4,68.03 CON-LEVEL2-I+/V+.8
I+5_3
  Top 0.254: IC402.19 118.3,100.93 120.95,103.58 CON-LEVEL3-I+/V+.8
I+5_4
  Top 0.254: IC402.3 86.55,102.43 85.4,103.58 CON-LEVEL4-I+/V+.8
I+7_1
  Top 0.254: IC401.20 116.26,65.87 118.42,68.03 CON-LEVEL1-I+/V+.10
I+7_2
  Top 0.254: IC401.4 84.51,66.37 82.85,68.03 CON-LEVEL2-I+/V+.10
I+7_3
  Top 0.254: IC402.20 116.26,101.43 118.42,103.58 CON-LEVEL3-I+/V+.10
I+7_4
  Top 0.254: IC402.4 84.51,101.93 82.85,103.58 CON-LEVEL4-I+/V+.10
I+9_1
  Top 0.254: IC401.21 114.22,66.37 115.88,68.03 CON-LEVEL1-I+/V+.12
I+9_2
  Top 0.254: IC401.5 82.47,65.87 80.31,68.03 CON-LEVEL2-I+/V+.12
I+9_3
  Top 0.254: IC402.21 114.22,101.93 115.88,103.58 CON-LEVEL3-I+/V+.12
I+9_4
  Top 0.254: IC402.5 82.47,101.43 80.31,103.58 CON-LEVEL4-I+/V+.12
I+11_1
  Top 0.254: IC401.22 112.18,66.87 113.33,68.03 CON-LEVEL1-I+/V+.14
I+11_2
  Top 0.254: IC401.6 80.43,65.37 77.78,68.03 CON-LEVEL2-I+/V+.14
I+11_3
  Top 0.254: IC402.22 112.18,102.43 113.33,103.58 CON-LEVEL3-I+/V+.14
I+11_4
  Top 0.254: IC402.6 80.43,100.93 77.78,103.58 CON-LEVEL4-I+/V+.14
I+13_1
  Top 0.254: IC401.23 110.14,67.37 110.8,68.03 CON-LEVEL1-I+/V+.16
I+13_2
  Top 0.254: IC401.7 78.39,64.87 75.23,68.03 CON-LEVEL2-I+/V+.16
I+13_3
  Top 0.254: IC402.23 110.14,102.93 110.8,103.58 CON-LEVEL3-I+/V+.16
I+13_4
  Top 0.254: IC402.7 78.39,100.43 75.23,103.58 CON-LEVEL4-I+/V+.16
I+15_1
  Top 0.254: IC401.24 108.1,67.87 108.25,68.03 CON-LEVEL1-I+/V+.18
I+15_2
  Top 0.254: IC401.8 76.35,64.37 72.69,68.03 CON-LEVEL2-I+/V+.18
I+15_3
  Top 0.254: IC402.24 108.1,103.43 108.25,103.58 CON-LEVEL3-I+/V+.18
I+15_4
  Top 0.254: IC402.8 76.35,99.93 72.69,103.58 CON-LEVEL4-I+/V+.18
I-  (via drill 0.25)
  Top 0.254: IC403.29 32.76,69.36 v33.01,69.61 | v33.01,105.17 32.76,104.92 IC404.29 | IC302.1 62.53,89.93 62.22,90.25 59.04,90.25 R316.2 58.73,88.66 34.91,88.66 I-.TP
  Bottom 0.254: v33.01,69.61 I-.TP | I-.TP v33.01,105.17 | I-.TP 33.01,90.89
  other vias: 33.01,90.57
I-2_1
  Top 0.254: IC403.17 56.02,64.37 59.68,68.03 CON-LEVEL1-I-/V-.4
I-2_2
  Top 0.254: IC403.1 24.27,67.87 24.12,68.03 CON-LEVEL2-I-/V-.4
I-2_3
  Top 0.254: IC404.17 56.02,99.93 59.68,103.58 CON-LEVEL3-I-/V-.4
I-2_4
  Top 0.254: IC404.1 24.27,103.43 24.12,103.58 CON-LEVEL4-I-/V-.4
I-4_1
  Top 0.254: IC403.18 53.98,64.87 57.14,68.03 CON-LEVEL1-I-/V-.6
I-4_2
  Top 0.254: IC403.2 22.23,67.37 21.58,68.03 CON-LEVEL2-I-/V-.6
I-4_3
  Top 0.254: IC404.18 53.98,100.43 57.14,103.58 CON-LEVEL3-I-/V-.6
I-4_4
  Top 0.254: IC404.2 22.23,102.93 21.58,103.58 CON-LEVEL4-I-/V-.6
I-6_1
  Top 0.254: IC403.19 51.94,65.37 54.6,68.03 CON-LEVEL1-I-/V-.8
I-6_2
  Top 0.254: IC403.3 20.19,66.87 19.04,68.03 CON-LEVEL2-I-/V-.8
I-6_3
  Top 0.254: IC404.19 51.94,100.93 54.6,103.58 CON-LEVEL3-I-/V-.8
I-6_4
  Top 0.254: IC404.3 20.19,102.43 19.04,103.58 CON-LEVEL4-I-/V-.8
I-8_1
  Top 0.254: IC403.20 49.9,65.87 52.06,68.03 CON-LEVEL1-I-/V-.10
I-8_2
  Top 0.254: IC403.4 18.15,66.37 16.5,68.03 CON-LEVEL2-I-/V-.10
I-8_3
  Top 0.254: IC404.20 49.9,101.43 52.06,103.58 CON-LEVEL3-I-/V-.10
I-8_4
  Top 0.254: IC404.4 18.15,101.93 16.5,103.58 CON-LEVEL4-I-/V-.10
I-10_1
  Top 0.254: IC403.21 47.86,66.37 49.52,68.03 CON-LEVEL1-I-/V-.12
I-10_2
  Top 0.254: IC403.5 16.11,65.87 13.96,68.03 CON-LEVEL2-I-/V-.12
I-10_3
  Top 0.254: IC404.21 47.86,101.93 49.52,103.58 CON-LEVEL3-I-/V-.12
I-10_4
  Top 0.254: IC404.5 16.11,101.43 13.96,103.58 CON-LEVEL4-I-/V-.12
I-12_1
  Top 0.254: IC403.22 45.82,66.87 46.98,68.03 CON-LEVEL1-I-/V-.14
I-12_2
  Top 0.254: IC403.6 14.07,65.37 11.42,68.03 CON-LEVEL2-I-/V-.14
I-12_3
  Top 0.254: IC404.22 45.82,102.43 46.98,103.58 CON-LEVEL3-I-/V-.14
I-12_4
  Top 0.254: IC404.6 14.07,100.93 11.42,103.58 CON-LEVEL4-I-/V-.14
I-14_1
  Top 0.254: IC403.23 43.78,67.37 44.44,68.03 CON-LEVEL1-I-/V-.16
I-14_2
  Top 0.254: IC403.7 12.03,64.87 8.88,68.03 CON-LEVEL2-I-/V-.16
I-14_3
  Top 0.254: IC404.23 43.78,102.93 44.44,103.58 CON-LEVEL3-I-/V-.16
I-14_4
  Top 0.254: IC404.7 12.03,100.43 8.88,103.58 CON-LEVEL4-I-/V-.16
I-16_1
  Top 0.254: IC403.24 41.74,67.87 41.9,68.03 CON-LEVEL1-I-/V-.18
I-16_2
  Top 0.254: IC403.8 9.99,64.37 6.34,68.03 CON-LEVEL2-I-/V-.18
I-16_3
  Top 0.254: IC404.24 41.74,103.43 41.9,103.58 CON-LEVEL3-I-/V-.18
I-16_4
  Top 0.254: IC404.8 9.99,99.93 6.34,103.58 CON-LEVEL4-I-/V-.18
N$1
  Top 0.61: PWR.2 D201.2
N$2  (via drill 1 pad 1.93)
  other vias: 9.2,90.89
N$3
  Top 0.254: T301.2 R302.1 | 68.25,59.71 IC301.16 68.56,59.45 SCL.TP R302.1 | 73.65,59.14 R302.1
N$4  (via drill 1 pad 1.93)
  other vias: 9.2,88.34
N$5
  Top 0.254: T302.2 R301.1 | 67.61,59.71 IC301.15 67.65,58.46 70.19,58.46 70.79,57.87 SDA.TP R301.1 | 73.65,55.64 R301.1
N$7
  Top 0.254: IC301.4 66.35,79.46 69.2,82.31 R303.1
N$8
  Top 0.254: 73.65,83.42 R304.1 74.6,85.49 VIN.TP | IC301.5 65.7,79.77 69.36,83.42 73.65,83.42 | 73.65,83.42 R303.2
N$9
  Top 0.254: IC302.7 70.16,86.76 | 70.16,86.76 R309.1 R304.2 | INST.TP 70.16,86.76
  Top 0.406: 70.16,88.66 IC302.7
N$10
  Top 0.254: R305.2 R306.1 IC303.1 79.4,91.2 1V65.TP
N$11
  Top 0.152: R308.1 60.95,91.52 61.58,90.89 67.61,90.89
  Top 0.254: IC302.5 67.61,90.89 70.16,90.89 71.75,89.3 R307.2
N$12
  Top 0.254: IC301.6 65.08,66.83 65.08,68.66 63.8,69.93 63.8,70.89 63.8,79.45 63.8,81.04 VOUT.TP C306.1
N$13
  Top 0.254: IC303.3 IC303.4 77.14,88.98 T1.TP R307.1
N$14  (via drill 0.25)
  Top 0.254: R309.2 73.97,86.44 | 73.65,86.44 73.33,86.44 R309.2 | R310.1 73.97,91.83 R310.1 v73.65,90.25 | IC302.6 v68.88,89.93 | v75.23,86.76 R309.2
  Bottom 0.254: v68.88,89.93 69.2,90.25 v73.65,90.25 74.92,90.25 75.23,89.93 v75.23,86.76
N$15
  Top 0.254: IC302.8 70.16,93.74 R313.1 R310.2
N$16
  Top 0.254: 62.53,93.11 IC302.14 62.53,95.01 59.04,95.01 | 59.04,95.01 R311.2 | R308.2 59.05,95.01 59.04,95.01
N$17
  Top 0.152: 68.25,94.69 68.25,91.84 67.93,91.52 64.12,91.52 63.8,91.84 IC302.13
  Top 0.254: R312.2 68.25,96.28 68.25,94.69 | R311.1 62.53,96.28 63.8,95.01 IC302.13
N$18
  Top 0.254: IC302.9 68.88,95.01 73.65,95.01 | 73.65,95.01 R313.2 | R312.1 73.65,95.01
N$19
  Top 0.254: C306.2 R314.1 HP.TP
N$20  (via drill 1 pad 1.93)
  other vias: 11.73,85.81
N$21  (via drill 1 pad 1.93)
  other vias: 11.73,88.34
N$22  (via drill 1 pad 1.93)
  other vias: 11.73,90.89
N$23  (via drill 1 pad 1.93)
  other vias: 14.27,93.42
N$24  (via drill 1 pad 1.93)
  other vias: 16.82,93.42
N$25  (via drill 1 pad 1.93)
  other vias: 19.36,93.42
N$26  (via drill 1 pad 1.93)
  other vias: 11.73,93.42
N$27  (via drill 1 pad 1.93)
  other vias: 9.2,93.42
N$28  (via drill 1 pad 1.93)
  other vias: 14.27,90.89
N$29  (via drill 1 pad 1.93)
  other vias: 16.82,90.89
N$30  (via drill 1 pad 1.93)
  other vias: 19.36,90.89
N$31  (via drill 1 pad 1.93)
  other vias: 107.94,90.89
N$32  (via drill 1 pad 1.93)
  other vias: 107.94,88.34
N$33  (via drill 1 pad 1.93)
  other vias: 21.89,90.89
N$34  (via drill 1 pad 1.93)
  other vias: 110.48,85.81
N$35  (via drill 1 pad 1.93)
  other vias: 110.48,88.34
N$36  (via drill 1 pad 1.93)
  other vias: 110.48,90.89
N$37  (via drill 1 pad 1.93)
  other vias: 113.02,93.42
N$38  (via drill 1 pad 1.93)
  other vias: 115.56,93.42
N$39  (via drill 1 pad 1.93)
  other vias: 118.1,93.42
N$40  (via drill 1 pad 1.93)
  other vias: 120.64,93.42
N$41  (via drill 1 pad 1.93)
  other vias: 123.18,93.42
N$42  (via drill 1 pad 1.93)
  other vias: 113.02,90.89
N$43  (via drill 1 pad 1.93)
  other vias: 115.56,90.89
N$44  (via drill 1 pad 1.93)
  other vias: 118.1,90.89
N$45  (via drill 1 pad 1.93)
  other vias: 120.64,90.89
N$46  (via drill 1 pad 1.93)
  other vias: 123.18,90.89
N$47  (via drill 1 pad 1.93)
  other vias: 113.02,88.34
N$48  (via drill 1 pad 1.93)
  other vias: 115.56,88.34
N$49  (via drill 1 pad 1.93)
  other vias: 118.1,88.34
N$50  (via drill 1 pad 1.93)
  other vias: 120.64,88.34
N$51  (via drill 1 pad 1.93)
  other vias: 123.18,88.34
N$52  (via drill 1 pad 1.93)
  other vias: 113.02,85.81
N$53  (via drill 1 pad 1.93)
  other vias: 115.56,85.81
N$54  (via drill 1 pad 1.93)
  other vias: 118.1,85.81
N$55  (via drill 1 pad 1.93)
  other vias: 120.64,85.81
N$56  (via drill 1 pad 1.93)
  other vias: 123.18,85.81
N$57  (via drill 1 pad 1.93)
  other vias: 24.44,90.89
N$58  (via drill 1 pad 1.93)
  other vias: 14.27,88.34
N$59  (via drill 1 pad 1.93)
  other vias: 16.82,88.34
N$60  (via drill 1 pad 1.93)
  other vias: 19.36,88.34
N$61  (via drill 1 pad 1.93)
  other vias: 21.89,88.34
N$62  (via drill 1 pad 1.93)
  other vias: 24.44,88.34
N$63  (via drill 1 pad 1.93)
  other vias: 14.27,85.81
N$64  (via drill 1 pad 1.93)
  other vias: 16.82,85.81
N$65  (via drill 1 pad 1.93)
  other vias: 19.36,85.81
N$66  (via drill 1 pad 1.93)
  other vias: 21.89,85.81
N$67  (via drill 1 pad 1.93)
  other vias: 81.59,24.21
N$68  (via drill 1 pad 1.93)
  other vias: 81.59,21.67
N$69  (via drill 1 pad 1.93)
  other vias: 84.12,19.13
N$70  (via drill 1 pad 1.93)
  other vias: 84.12,21.67
N$71  (via drill 1 pad 1.93)
  other vias: 84.12,29.29
N$72  (via drill 1 pad 1.93)
  other vias: 81.59,29.29
N$73  (via drill 1 pad 1.93)
  other vias: 89.2,26.75
N$74  (via drill 1 pad 1.93)
  other vias: 91.75,26.75
N$75  (via drill 1 pad 1.93)
  other vias: 94.28,26.75
N$76  (via drill 1 pad 1.93)
  other vias: 96.83,26.75
N$78  (via drill 1 pad 1.93)
  other vias: 89.2,24.21
N$79  (via drill 1 pad 1.93)
  other vias: 91.75,24.21
N$80  (via drill 1 pad 1.93)
  other vias: 94.28,24.21
N$81  (via drill 1 pad 1.93)
  other vias: 96.83,24.21
N$82  (via drill 1 pad 1.93)
  other vias: 86.66,21.67
N$83  (via drill 1 pad 1.93)
  other vias: 89.2,21.67
N$84  (via drill 1 pad 1.93)
  other vias: 91.75,21.67
N$85  (via drill 1 pad 1.93)
  other vias: 94.28,21.67
N$86  (via drill 1 pad 1.93)
  other vias: 96.83,21.67
N$87  (via drill 1 pad 1.93)
  other vias: 86.66,19.13
N$88  (via drill 1 pad 1.93)
  other vias: 89.2,19.13
N$89  (via drill 1 pad 1.93)
  other vias: 91.75,19.13
N$90
  Top 0.254: MCLK.TP 62.22,62.63 63.75,64.16 IC301.8
N$93  (via drill 1 pad 1.93)
  other vias: 71.42,26.75
N$94  (via drill 1 pad 1.93)
  other vias: 73.97,26.75
N$95  (via drill 1 pad 1.93)
  other vias: 76.5,26.75
N$96  (via drill 1 pad 1.93)
  other vias: 79.05,24.21
N$99  (via drill 1 pad 1.93)
  other vias: 71.42,21.67
N$100  (via drill 1 pad 1.93)
  other vias: 73.97,21.67
N$101  (via drill 1 pad 1.93)
  other vias: 76.5,21.67
N$102  (via drill 1 pad 1.93)
  other vias: 79.05,21.67
N$107  (via drill 1 pad 1.93)
  other vias: 79.05,19.13
N$109  (via drill 1 pad 1.93)
  other vias: 71.42,24.21
N$110  (via drill 1 pad 1.93)
  other vias: 73.97,24.21
N$111  (via drill 1 pad 1.93)
  other vias: 76.5,24.21
N$112  (via drill 1 pad 1.93)
  other vias: 79.05,29.29
N$114  (via drill 1 pad 1.93)
  other vias: 71.42,29.29
N$115  (via drill 1 pad 1.93)
  other vias: 73.97,29.29
N$116  (via drill 1 pad 1.93)
  other vias: 76.5,29.29
N$117  (via drill 1 pad 1.93)
  other vias: 96.83,29.29
N$118  (via drill 1 pad 1.93)
  other vias: 86.66,29.29
N$119  (via drill 1 pad 1.93)
  other vias: 89.2,29.29
N$120  (via drill 1 pad 1.93)
  other vias: 91.75,29.29
N$121  (via drill 1 pad 1.93)
  other vias: 94.28,29.29
N$124  (via drill 1 pad 1.93)
  other vias: 81.59,34.37
N$125  (via drill 1 pad 1.93)
  other vias: 84.12,31.83
N$126  (via drill 1 pad 1.93)
  other vias: 84.12,34.37
N$128  (via drill 1 pad 1.93)
  other vias: 86.66,36.91
N$129  (via drill 1 pad 1.93)
  other vias: 89.2,36.91
N$130  (via drill 1 pad 1.93)
  other vias: 91.75,36.91
N$131  (via drill 1 pad 1.93)
  other vias: 94.28,36.91
N$132  (via drill 1 pad 1.93)
  other vias: 96.83,36.91
N$133  (via drill 1 pad 1.93)
  other vias: 86.66,34.37
N$134  (via drill 1 pad 1.93)
  other vias: 89.2,34.37
N$135  (via drill 1 pad 1.93)
  other vias: 91.75,34.37
N$136  (via drill 1 pad 1.93)
  other vias: 94.28,34.37
N$137  (via drill 1 pad 1.93)
  other vias: 96.83,34.37
N$138  (via drill 1 pad 1.93)
  other vias: 86.66,31.83
N$139  (via drill 1 pad 1.93)
  other vias: 89.2,31.83
N$140  (via drill 1 pad 1.93)
  other vias: 91.75,31.83
N$141  (via drill 1 pad 1.93)
  other vias: 94.28,31.83
N$142  (via drill 1 pad 1.93)
  other vias: 96.83,31.83
N$145  (via drill 1 pad 1.93)
  other vias: 71.42,34.37
N$146  (via drill 1 pad 1.93)
  other vias: 73.97,34.37
N$147  (via drill 1 pad 1.93)
  other vias: 76.5,34.37
N$148  (via drill 1 pad 1.93)
  other vias: 79.05,34.37
N$150  (via drill 1 pad 1.93)
  other vias: 71.42,31.83
N$151  (via drill 1 pad 1.93)
  other vias: 73.97,31.83
N$152  (via drill 1 pad 1.93)
  other vias: 76.5,31.83
N$153  (via drill 1 pad 1.93)
  other vias: 79.05,31.83
N$154  (via drill 1 pad 1.93)
  other vias: 84.12,26.75
N$155  (via drill 1 pad 1.93)
  other vias: 86.66,26.75
N$156  (via drill 1 pad 1.93)
  other vias: 84.12,24.21
N$157  (via drill 1 pad 1.93)
  other vias: 86.66,24.21
N$158  (via drill 1 pad 1.93)
  other vias: 79.05,26.75
N$159  (via drill 1 pad 1.93)
  other vias: 81.59,26.75
RX1  (via drill 1 pad 1.93)
  Bottom 0.254: v96.83,19.13 105.4,19.13 109.53,15 MEGA_CON4.6
SCL  (via drill 0.25)
  Top 0.254: T301.3 78.19,59.04 78.73,58.5 111.75,58.5 114.92,55.33 114.92,53.42 v115.88,52.47
  Bottom 0.254: v115.88,52.47 115.88,3.89 MEGA_CON4.8
SDA  (via drill 0.25)
  Top 0.254: T302.3 78.19,57.33 78.73,57.87 111.43,57.87 114.29,55.01 114.29,53.42 v113.33,52.47
  Bottom 0.254: v113.33,52.47 113.33,3.89 MEGA_CON4.7
TX1  (via drill 1 pad 1.93)
  Bottom 0.254: v94.28,19.13 94.28,18.18 94.92,17.54 98.41,17.54 99.37,18.5 105.08,18.5 108.89,14.68 108.89,4.53 MEGA_CON4.5
V+  (via drill 0.25)
  Top 0.254: v99.05,120.73 99.12,120.66 IC502.29 | IC501.29 99.12,84.6 100,85.49 v102.22,85.49 | IC302.10 67.61,97.55 68.25,98.19 94.6,98.19 96.83,95.97 100.64,95.97 102.22,94.38 V+.TP
  Bottom 0.254: v102.22,85.49 V+.TP 102.22,120.09 101.59,120.73 v99.05,120.73
  other vias: 102.22,90.57
V+1_1
  Top 0.254: IC501.24 121.43,82.79 126.03,78.19 CON-LEVEL1-I+/V+.3
V+1_2
  Top 0.254: IC501.8 91.58,79.29 90.47,78.19 CON-LEVEL2-I+/V+.3
V+1_3
  Top 0.254: IC502.24 121.43,118.35 126.03,113.75 CON-LEVEL3-I+/V+.3
V+1_4
  Top 0.254: IC502.8 91.58,114.85 90.47,113.75 CON-LEVEL4-I+/V+.3
V+3_1
  Top 0.254: IC501.23 119.39,82.29 123.5,78.19 CON-LEVEL1-I+/V+.5
V+3_2
  Top 0.254: IC501.7 89.54,79.79 87.94,78.19 CON-LEVEL2-I+/V+.5
V+3_3
  Top 0.254: IC502.23 119.39,117.85 123.5,113.75 CON-LEVEL3-I+/V+.5
V+3_4
  Top 0.254: IC502.7 89.54,115.35 87.94,113.75 CON-LEVEL4-I+/V+.5
V+5_1
  Top 0.254: IC501.22 117.35,81.79 120.95,78.19 CON-LEVEL1-I+/V+.7
V+5_2
  Top 0.254: IC501.6 87.5,80.29 85.4,78.19 CON-LEVEL2-I+/V+.7
V+5_3
  Top 0.254: IC502.22 117.35,117.35 120.95,113.75 CON-LEVEL3-I+/V+.7
V+5_4
  Top 0.254: IC502.6 87.5,115.85 85.4,113.75 CON-LEVEL4-I+/V+.7
V+7_1
  Top 0.254: IC501.21 115.31,81.29 118.42,78.19 CON-LEVEL1-I+/V+.9
V+7_2
  Top 0.254: IC501.5 85.46,80.79 82.85,78.19 CON-LEVEL2-I+/V+.9
V+7_3
  Top 0.254: IC502.21 115.31,116.85 118.42,113.75 CON-LEVEL3-I+/V+.9
V+7_4
  Top 0.254: IC502.5 85.46,116.35 82.85,113.75 CON-LEVEL4-I+/V+.9
V+9_1
  Top 0.254: IC501.20 113.27,80.79 115.88,78.19 CON-LEVEL1-I+/V+.11
V+9_2
  Top 0.254: IC501.4 83.42,81.29 80.31,78.19 CON-LEVEL2-I+/V+.11
V+9_3
  Top 0.254: IC502.20 113.27,116.35 115.88,113.75 CON-LEVEL3-I+/V+.11
V+9_4
  Top 0.254: IC502.4 83.42,116.85 80.31,113.75 CON-LEVEL4-I+/V+.11
V+11_1
  Top 0.254: IC501.19 111.23,80.29 113.33,78.19 CON-LEVEL1-I+/V+.13
V+11_2
  Top 0.254: IC501.3 81.38,81.79 77.78,78.19 CON-LEVEL2-I+/V+.13
V+11_3
  Top 0.254: IC502.19 111.23,115.85 113.33,113.75 CON-LEVEL3-I+/V+.13
V+11_4
  Top 0.254: IC502.3 81.38,117.35 77.78,113.75 CON-LEVEL4-I+/V+.13
V+13_1
  Top 0.254: IC501.18 109.19,79.79 110.8,78.19 CON-LEVEL1-I+/V+.15
V+13_2
  Top 0.254: IC501.2 79.34,82.29 75.23,78.19 CON-LEVEL2-I+/V+.15
V+13_3
  Top 0.254: IC502.18 109.19,115.35 110.8,113.75 CON-LEVEL3-I+/V+.15
V+13_4
  Top 0.254: IC502.2 79.34,117.85 75.23,113.75 CON-LEVEL4-I+/V+.15
V+15_1
  Top 0.254: IC501.17 107.15,79.29 108.25,78.19 CON-LEVEL1-I+/V+.17
V+15_2
  Top 0.254: IC501.1 77.3,82.79 72.69,78.19 CON-LEVEL2-I+/V+.17
V+15_3
  Top 0.254: IC502.17 107.15,114.85 108.25,113.75 CON-LEVEL3-I+/V+.17
V+15_4
  Top 0.254: IC502.1 77.3,118.35 72.69,113.75 CON-LEVEL4-I+/V+.17
V-  (via drill 0.25)
  Top 0.254: IC302.12 65.08,97.55 64.44,98.19 v35.87,98.19 | IC504.29 32.76,120.66 v32.69,120.73 | IC503.29 32.76,84.6 33.33,85.17 v35.87,85.17
  Bottom 0.254: v32.69,120.73 35.23,120.73 35.87,120.09 v35.87,98.19 V-.TP v35.87,85.17
  other vias: 35.87,90.57
V-2_1
  Top 0.254: IC503.24 55.07,82.79 59.68,78.19 CON-LEVEL1-I-/V-.3
V-2_2
  Top 0.254: IC503.8 25.23,79.29 24.12,78.19 CON-LEVEL2-I-/V-.3
V-2_3
  Top 0.254: IC504.24 55.07,118.35 59.68,113.75 CON-LEVEL3-I-/V-.3
V-2_4
  Top 0.254: IC504.8 25.23,114.85 24.12,113.75 CON-LEVEL4-I-/V-.3
V-4_1
  Top 0.254: IC503.23 53.03,82.29 57.14,78.19 CON-LEVEL1-I-/V-.5
V-4_2
  Top 0.254: IC503.7 23.19,79.79 21.58,78.19 CON-LEVEL2-I-/V-.5
V-4_3
  Top 0.254: IC504.23 53.03,117.85 57.14,113.75 CON-LEVEL3-I-/V-.5
V-4_4
  Top 0.254: IC504.7 23.19,115.35 21.58,113.75 CON-LEVEL4-I-/V-.5
V-6_1
  Top 0.254: IC503.22 50.99,81.79 54.6,78.19 CON-LEVEL1-I-/V-.7
V-6_2
  Top 0.254: IC503.6 21.14,80.29 19.04,78.19 CON-LEVEL2-I-/V-.7
V-6_3
  Top 0.254: IC504.22 50.99,117.35 54.6,113.75 CON-LEVEL3-I-/V-.7
V-6_4
  Top 0.254: IC504.6 21.14,115.85 19.04,113.75 CON-LEVEL4-I-/V-.7
V-8_1
  Top 0.254: IC503.21 48.95,81.29 52.06,78.19 CON-LEVEL1-I-/V-.9
V-8_2
  Top 0.254: IC503.5 19.11,80.79 16.5,78.19 CON-LEVEL2-I-/V-.9
V-8_3
  Top 0.254: IC504.21 48.95,116.85 52.06,113.75 CON-LEVEL3-I-/V-.9
V-8_4
  Top 0.254: IC504.5 19.11,116.35 16.5,113.75 CON-LEVEL4-I-/V-.9
V-10_1
  Top 0.254: IC503.20 46.91,80.79 49.52,78.19 CON-LEVEL1-I-/V-.11
V-10_2
  Top 0.254: IC503.4 17.07,81.29 13.96,78.19 CON-LEVEL2-I-/V-.11
V-10_3
  Top 0.254: IC504.20 46.91,116.35 49.52,113.75 CON-LEVEL3-I-/V-.11
V-10_4
  Top 0.254: IC504.4 17.07,116.85 13.96,113.75 CON-LEVEL4-I-/V-.11
V-12_1
  Top 0.254: IC503.19 44.87,80.29 46.98,78.19 CON-LEVEL1-I-/V-.13
V-12_2
  Top 0.254: IC503.3 15.02,81.79 11.42,78.19 CON-LEVEL2-I-/V-.13
V-12_3
  Top 0.254: IC504.19 44.87,115.85 46.98,113.75 CON-LEVEL3-I-/V-.13
V-12_4
  Top 0.254: IC504.3 15.02,117.35 11.42,113.75 CON-LEVEL4-I-/V-.13
V-14_1
  Top 0.254: IC503.18 42.83,79.79 44.44,78.19 CON-LEVEL1-I-/V-.15
V-14_2
  Top 0.254: IC503.2 12.98,82.29 8.88,78.19 CON-LEVEL2-I-/V-.15
V-14_3
  Top 0.254: IC504.18 42.83,115.35 44.44,113.75 CON-LEVEL3-I-/V-.15
V-14_4
  Top 0.254: IC504.2 12.98,117.85 8.88,113.75 CON-LEVEL4-I-/V-.15
V-16_1
  Top 0.254: IC503.17 40.79,79.29 41.9,78.19 CON-LEVEL1-I-/V-.17
V-16_2
  Top 0.254: IC503.1 10.95,82.79 6.34,78.19 CON-LEVEL2-I-/V-.17
V-16_3
  Top 0.254: IC504.17 40.79,114.85 41.9,113.75 CON-LEVEL3-I-/V-.17
V-16_4
  Top 0.254: IC504.1 10.95,118.35 6.34,113.75 CON-LEVEL4-I-/V-.17
VIN_MEGA  (via drill 0.25)
  Top 0.406: 16.16,17.69 16.16,19.43 v16.18,19.45
  Top 0.61: D201.1 16.16,17.69 16.16,20.74 11.73,25.16 IC201.23 IC201.22
  Bottom 0.406: v16.18,19.45 17.45,19.45 21.58,23.57 21.58,39.45 25.07,42.94 71.42,42.94 73.97,45.48 MEGA_CON1.1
